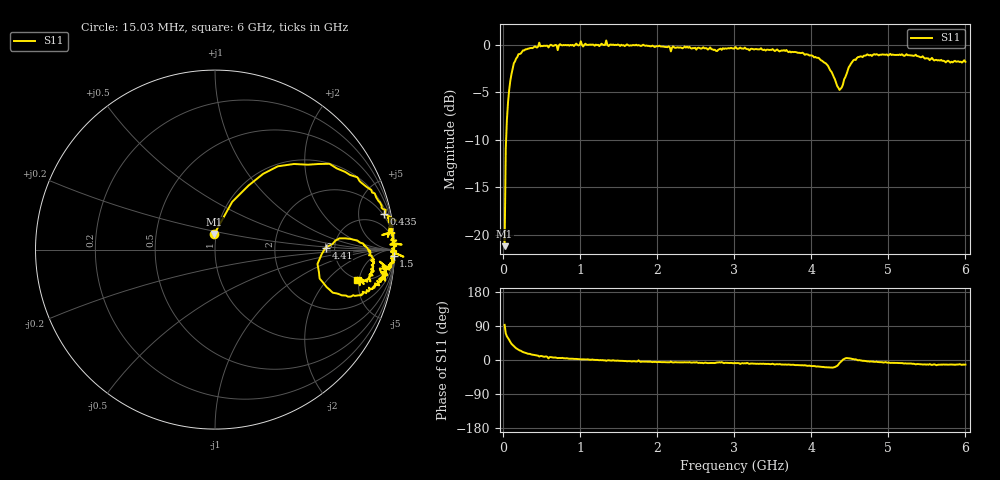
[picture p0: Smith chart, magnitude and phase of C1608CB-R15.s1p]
!	Network	Analyzer	HP8753E.07.74:	Oct	30	2002	Serial	No.	JP38451487
!	Hewlett-Packard
!	7	Sep	2009	10:01:29
!	Frequency	S11
#	HZ	S	RI	R	50
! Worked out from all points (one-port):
!   400 points, 15.03 MHz to 6 GHz, reference 50 ohm
!   lowest |S11| = -21.2 dB at 15.03 MHz (marker M1), VSWR 1.19, Z = 48.9 + j8.55 ohm
!   |S11| at or under -10 dB: start of sweep to 34.77 MHz
!   S11 on the Smith chart (normalised r, x): 15.03 MHz: 0.98, +0.17; 435 MHz: 1.66, +9.29; 1.5 GHz: 6, -54; 4.41 GHz: 4.22, +0.16; 6 GHz: 4.74, -4.74
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1.502992e7  -0.00412 0.0868
3.002985e7  0.0957 0.266
6.00297e7  0.268 0.422
9.002955e7  0.44 0.477
1.95029e8  0.793 0.403
4.350278e8  0.943 0.199
4.650277e8  1.01 0.162
5.550272e8  0.972 0.163
5.850271e8  0.963 0.07
6.150269e8  0.988 0.134
7.650262e8  0.985 0.097
1.005025e9  1.04 0.0281
1.035025e9  0.976 0.0283
1.245024e9  0.981 -0.00977
1.335023e9  1.05 -0.0397
1.365023e9  0.981 -0.0126
1.500022e9  0.995 -0.0363
1.515022e9  0.982 -0.0371
2.265019e9  0.962 -0.102
3.015015e9  0.961 -0.141
3.765011e9  0.891 -0.197
4.230009e9  0.707 -0.255
4.335008e9  0.583 -0.161
4.410008e9  0.617 0.0116
4.515007e9  0.793 0.0508
4.725006e9  0.886 -0.0572
5.265004e9  0.867 -0.146
6e9  0.793 -0.171
